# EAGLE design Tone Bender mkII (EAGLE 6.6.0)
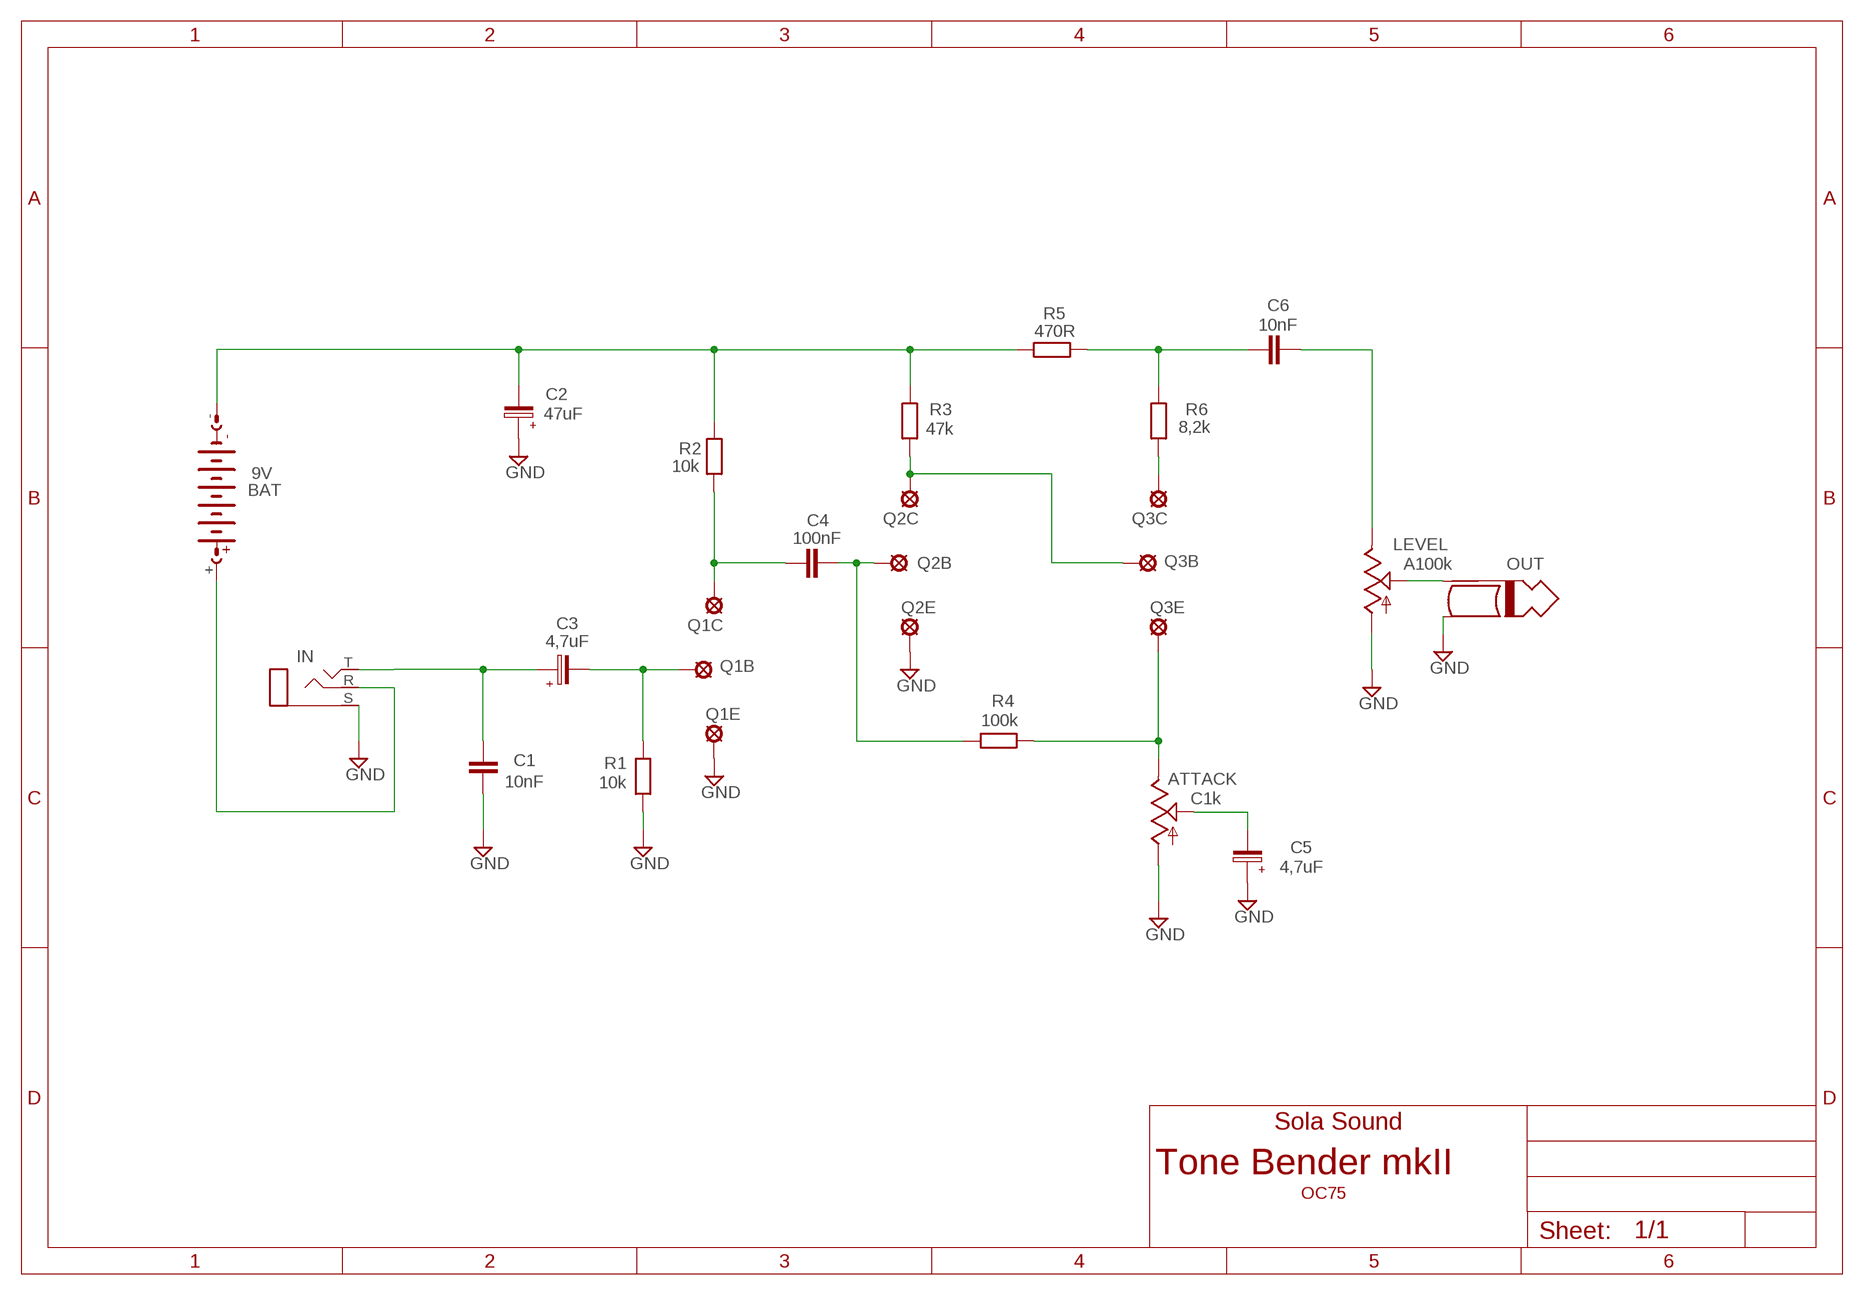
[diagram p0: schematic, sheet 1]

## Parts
ATTACK  C1k  9MM_SNAP-IN_POT_  [9MM_SNAP-IN_POT]
BAT  9V  AB9V  [AB9V]
C1  10nF  C10/4  [C10B4]
C2  47uF  063-EU  [063_025]
C3  4,7uF  050-EU  [050_020]
C4  100nF  C10/4  [C10B4]
C5  4,7uF  050-EU  [050_020]
C6  10nF  C10/4  [C10B4]
IN  STEREOPADS  [STEREO_PADS]
LEVEL  A100k  9MM_SNAP-IN_POT_  [9MM_SNAP-IN_POT]
OUT  MONO_PLUG  [TWO_PADS]
Q1B  LSP10  [LSP10]
Q1C  LSP10  [LSP10]
Q1E  LSP10  [LSP10]
Q2B  LSP10  [LSP10]
Q2C  LSP10  [LSP10]
Q2E  LSP10  [LSP10]
Q3B  LSP10  [LSP10]
Q3C  LSP10  [LSP10]
Q3E  LSP10  [LSP10]
R1  10k  6MM-EU3  [R0207/3]
R2  10k  6MM-EU3  [R0207/3]
R3  47k  6MM-EU3  [R0207/3]
R4  100k  6MM-EU3  [R0207/3]
R5  470R  6MM-EU3  [R0207/3]
R6  8,2k  6MM-EU3  [R0207/3]

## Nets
GND: ATTACK.1(A) C1.1 C2.+ C5.+ IN.S(R) LEVEL.1(A) OUT.SLEEVE Q1E.MP Q2E.MP R1.1
N$1: C6.1 R5.1 R6.1
N$2: C4.1 Q1C.MP R2.1
N$3: Q2C.MP Q3B.MP R3.1
N$4: Q3C.MP R6.2
N$5: ATTACK.3(E) Q3E.MP R4.2
N$6: C3.- Q1B.MP R1.2
N$7: C6.2 LEVEL.3(E)
N$8: LEVEL.2(S) OUT.TIP
N$9: C4.2 Q2B.MP R4.1
N$10: C1.2 C3.+ IN.T
N$11: ATTACK.2(S) C5.-
N$18: BAT.- C2.- R2.2 R3.2 R5.2
N$19: BAT.+ IN.R(S)

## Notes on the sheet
- Sola Sound
- OC75

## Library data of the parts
ATTACK LEVEL = MusicThingModular:9MM_SNAP-IN_POT: 9mm vertical snap-in pot, Alpha / Panasonic style
BAT = Battery:AB9V: 9-V BATTERY CLIP
C1 C4 C6 = capacitor-wima:C: CAPACITOR
C2 = Elektrolyytit:063-EU
C3 C5 = Elektrolyytit:050-EU
IN = gm-jacks:STEREO: Stereo (TRS) 1/4" Phone Jack often use for the input jack to disconnect battery when there is no plug in the jack also called TRS or tip-ring-sleeve jack
OUT = gm-jacks:MONO_PLUG
Q1B Q1C Q1E Q2B Q2C Q2E Q3B Q3C Q3E = Padit:LSP10: SOLDER PAD
R1-R6 = Vastukset:6MM-EU: 6mm Resistors (European schematic symbol)

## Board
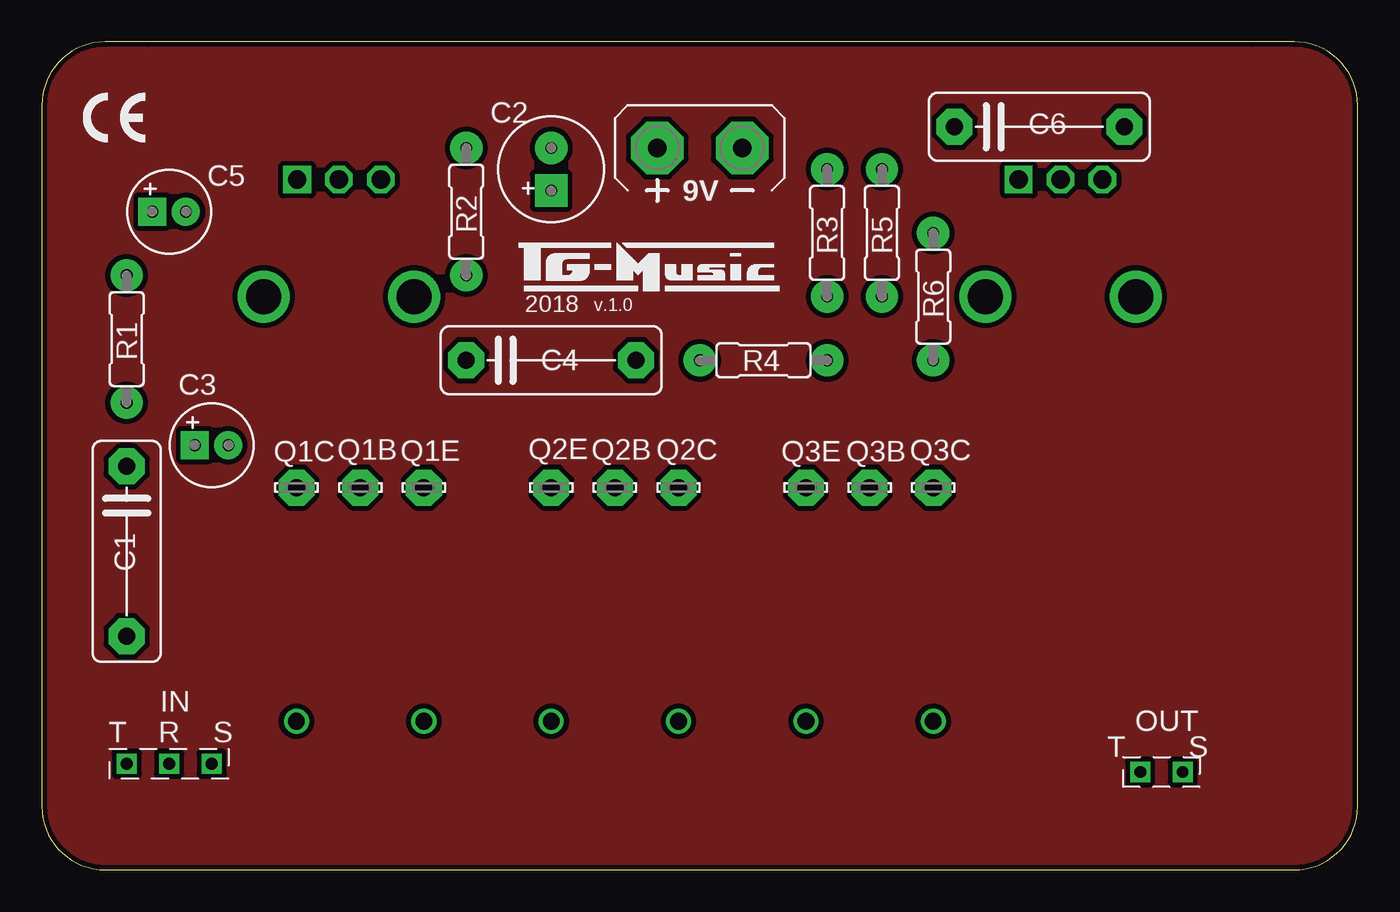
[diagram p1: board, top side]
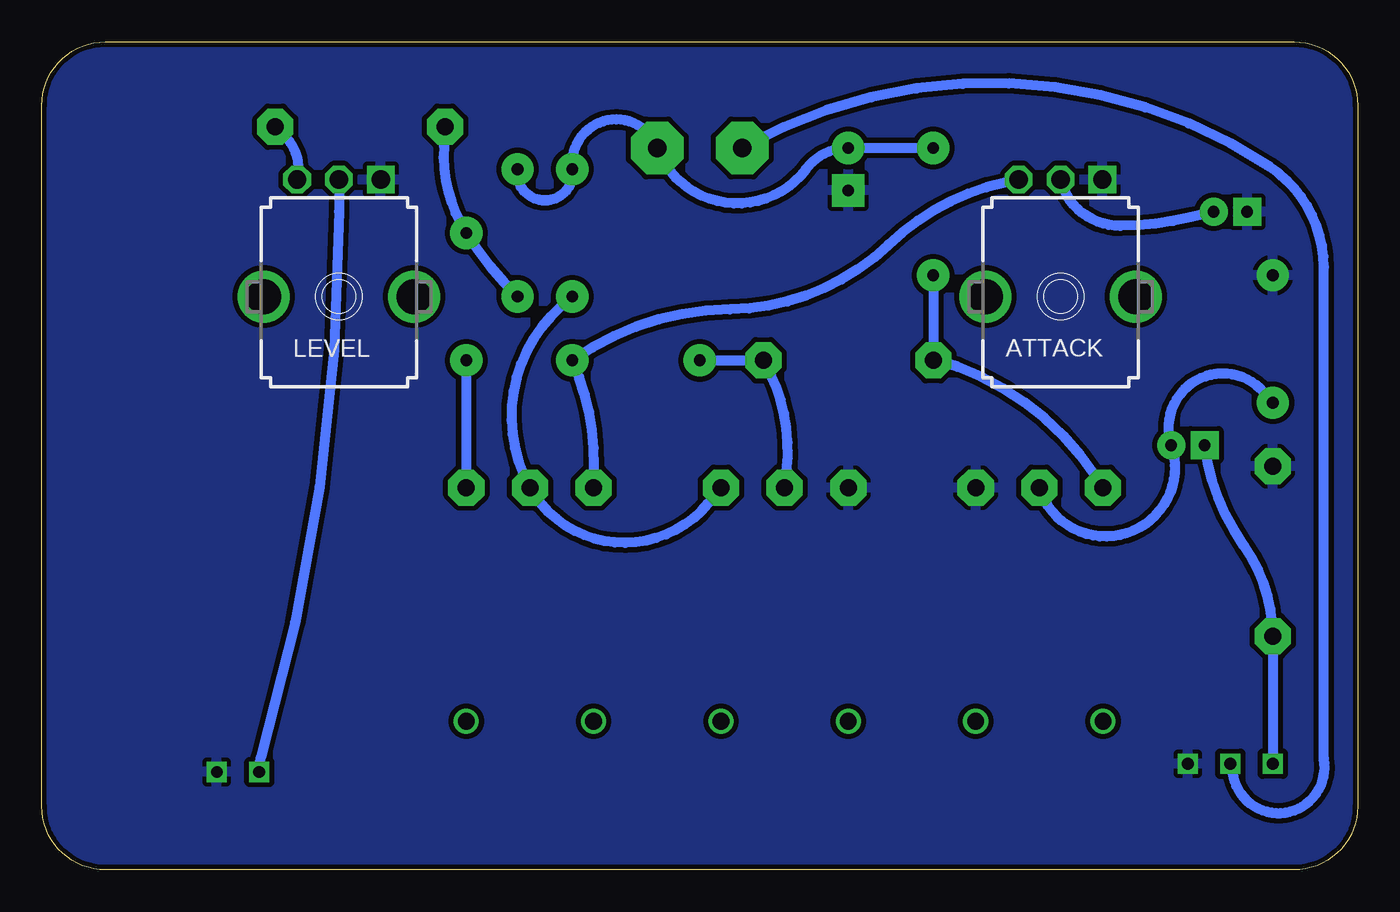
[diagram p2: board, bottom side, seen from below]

Size 78.74 x 49.53 mm. Coordinates in mm from the lower left corner, seen from the top.
Outline: 0,3.81 arc90 3.81,0 6.35,0 73.66,0 74.93,0 arc90 78.74,3.81 78.74,45.72 arc90 74.93,49.53 72.39,49.53 6.35,49.53 3.81,49.53 arc90 0,45.72 0,3.81
Copper layers (1*16): Top 0.035mm / dielectric 1.5mm / Bottom 0.035mm
Design rules "ITEADstudio": minimum track width 10mil, minimum drill 12mil, track to track 12mil, track to pad 12mil, pad to pad 12mil, via to via 12mil, smd to smd 0mil, copper to edge 12mil, drill to drill 12mil, minimum pad ring 10mil, minimum via ring 6mil, stop-mask expansion 4mil, vias tented up to drill 100mil, thermal gap 10mil

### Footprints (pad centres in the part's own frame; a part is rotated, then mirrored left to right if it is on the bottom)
9MM_SNAP-IN_POT = drill 1.1 square: 1 -2.5,-7 | drill 1.1 octagon: 2 0,-7; 3 2.5,-7 | drill 2.1 pad 2.794: CHASSIS1 -4.5,0; CHASSIS2 4.5,0
AB9V = drill 1.118 pad 3.15 octagon: + 0,2.54; - 0,-2.54
C10B4 = drill 1.016 pad 2.159 octagon: 1 -5.08,0; 2 5.08,0
063_025 = drill 0.7 pad 1.93 square: + -1.27,0 | drill 0.7 pad 1.93: - 1.27,0
050_020 = drill 0.7 pad 1.676 square: + -1,0 | drill 0.7 pad 1.676: - 1,0
STEREO_PADS = drill 0.7 square: R 0,0; S -2.54,0; T 2.54,0
TWO_PADS = drill 0.7 square: SLEEVE -1.27,0; TIP 1.27,0
LSP10 = drill 1.016 pad 2.159 octagon: MP 0,0
R0207/3 = drill 0.7 pad 1.93: 1 -3.81,0; 2 3.81,0

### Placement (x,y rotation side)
ATTACK  17.78,34.29 180 bottom
BAT  39.37,43.18 90 top
C1  5.08,19.05 270 top
C2  30.48,41.91 90 top
C3  10.16,25.4 0 top
C4  30.48,30.48 0 top
C5  7.62,39.37 0 top
C6  59.69,44.45 0 top
IN  7.62,6.35 180 top
LEVEL  60.96,34.29 180 bottom
OUT  67,5.86 180 top
Q1B  19.05,22.86 0 top
Q1C  15.24,22.86 0 top
Q1E  22.86,22.86 0 top
Q2B  34.29,22.86 0 top
Q2C  38.1,22.86 0 top
Q2E  30.48,22.86 0 top
Q3B  49.53,22.86 0 top
Q3C  53.34,22.86 0 top
Q3E  45.72,22.86 0 top
R1  5.08,31.75 270 top
R2  25.4,39.37 90 top
R3  46.99,38.1 90 top
R4  43.18,30.48 0 top
R5  50.27,38.1 90 top
R6  53.34,34.29 270 top

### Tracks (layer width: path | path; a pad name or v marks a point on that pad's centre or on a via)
GND
  pour Bottom: 0,3.81 0,45.72 arc-90 3.81,49.53 74.93,49.53 arc-90 78.74,45.72 78.74,3.81 arc-90 74.93,0 3.81,0 arc-90
N$1
  Bottom 0.61: C6.1 54.68,43.3 arc-36 R6.1 arc-13 R5.1
N$2
  Bottom 0.61: R2.1 25.4,30.54 | 25.4,30.54 C4.1 | Q1C.MP 15.71,23.57 arc-42 25.4,30.54
N$3
  Bottom 0.61: Q2C.MP 38.87,21.92 arc111 Q3B.MP arc78 47.67,33.7 R3.1
N$4
  Bottom 0.61: R6.2 Q3C.MP
N$5
  Bottom 0.61: Q3E.MP 45.7,24.15 arc-25 R4.2 arc34 37.56,33.53 arc-43 28.09,37.4 arc31 21.12,41.1 ATTACK.3
N$6
  Bottom 0.61: R1.2 5.6,28.55 arc-158 C3.- arc181 Q1B.MP
N$7
  Bottom 0.61: C6.2 64.29,44 arc60 LEVEL.3
N$8
  Bottom 0.61: LEVEL.2 60.96,39.37 arc16 65.61,6.79 arc-19 OUT.TIP
N$9
  Bottom 0.61: R4.1 C4.2 arc37 34.17,23.86 Q2B.MP
N$10
  Bottom 0.61: C3.+ arc-28 6.81,19.39 arc35 C1.2 IN.T
N$11
  Bottom 0.61: C5.- 9.99,39.04 arc13 14.21,38.52 arc76 ATTACK.2
N$12  (via drill 1)
  other vias: 15.24,8.89
N$13  (via drill 1)
  other vias: 30.48,8.89
N$14  (via drill 1)
  other vias: 22.86,8.89
N$15  (via drill 1)
  other vias: 45.72,8.89
N$16  (via drill 1)
  other vias: 38.1,8.89
N$17  (via drill 1)
  other vias: 53.34,8.89
N$18
  Bottom 0.61: R5.2 arc-195 R3.2 arc167 BAT.- arc-123 33.02,41.91 arc53 C2.- R2.2
N$19
  Bottom 0.61: IN.R 7.44,5.55 arc-178 2.03,6.65 2.03,36.05 arc-57 5.25,42.03 arc-63 BAT.+
N$20
  pour Top: 0,2.54 0,45.72 arc-90 3.81,49.53 74.93,49.53 arc-90 78.74,45.72 78.74,3.81 arc-90 74.93,0 2.54,0 arc-90

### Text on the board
tNames: 2018 | v.1.0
